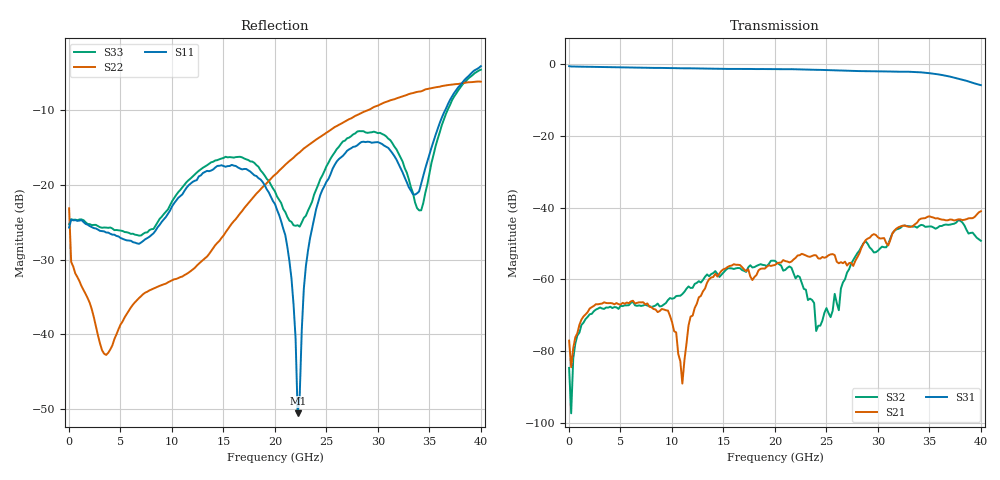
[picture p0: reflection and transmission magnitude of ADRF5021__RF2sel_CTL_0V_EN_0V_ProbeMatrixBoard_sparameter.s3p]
! Device:  ADRF5021
! Description: SOI MMIC SPDT Non-Reflective Switch
! Frequency:  9 kHz -  30 GHz
! Ports:
! 	RFC	= Port 1
!	RF1	= Port 2
!	RF2	= Port 3
! Vdd:  +3.3 Volt
! Vss:  -2.5 Volt
! Control:  0/+3.3 Volt
! State:  RF2 Selected (Vctl= 0 V, Ven= 0 V)
! Data:  The device was measured using G-S-G Probes on a matrix board.
!  Data was collected using an calibrated 4 port network analyzer.
!  The reference plane is the package pins of ADRF5021 switch.
! Note:  Analog Devices supplies this data as a sample of measured data at the package pin
!  for this product.  Your particular data for this product may vary.
!  Data was taken at 25 degrees C.
!  Analog Devices reserves the right to change this data at anytime.
# GHZ S DB R 50.0
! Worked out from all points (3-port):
!   201 points, 10 MHz to 40.01 GHz, reference 50 ohm
!   strongest paths, dB at 10 MHz, 10.01 GHz, 20.01 GHz, 30.01 GHz, 40.01 GHz:
!     S31: -0.6, -1.1, -1.4, -2.0, -5.9
!     S21: -77.1, -71.9, -56.0, -48.3, -41.0
!     S32: -84.7, -65.5, -54.9, -52.0, -49.3
!   lowest |S11| = -50.6 dB at 22.21 GHz (marker M1), VSWR 1.01, Z = 49.7 + j0.138 ohm
!   |S11| at or under -10 dB: start of sweep to 36.55 GHz
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0.01  -25.73 -14.1  -79.45 56.9  -0.58 0.3
      -77.11 -16.3  -23.15 79.6  -78.50 51.2
      -0.58 0.3  -84.72 -57.5  -25.27 -9.6
3.41  -26.24 -51.2  -66.72 32.8  -0.83 -40.4
      -66.43 34.1  -42.60 -166.9  -68.12 13.7
      -0.83 -40.4  -68.26 14.0  -25.72 -55.7
8.61  -25.68 -51.3  -69.35 19.9  -1.06 -100.7
      -69.15 18.3  -33.62 -94.7  -67.46 -56.8
      -1.05 -100.6  -66.78 -54.3  -24.99 -57.9
11.21  -20.83 -57.1  -81.36 -124.6  -1.18 -130.7
       -82.62 -137.9  -32.08 -73.6  -63.39 -109.7
       -1.18 -130.6  -63.49 -110.7  -19.99 -61.7
20.01  -22.58 -149.7  -55.96 102.3  -1.40 126.5
       -56.02 102.5  -18.66 -37.4  -54.87 65.2
       -1.40 126.6  -54.85 65.4  -20.90 -127.0
22.21  -50.57 152.2  -53.37 96.8  -1.46 99.7
       -53.37 96.4  -15.87 -41.9  -59.17 32.6
       -1.46 99.8  -59.02 32.0  -25.41 -87.7
25.61  -17.85 -38.1  -53.12 78.5  -1.75 57.9
       -52.99 78.5  -12.45 -53.2  -68.02 -114.2
       -1.73 58.0  -68.80 -110.3  -16.06 -53.0
28.81  -14.29 -72.4  -49.02 114.6  -1.97 18.9
       -49.10 115.7  -10.14 -66.0  -49.43 128.1
       -1.97 19.1  -49.39 129.3  -13.00 -81.1
34.21  -19.84 -41.3  -43.13 77.8  -2.31 -54.3
       -43.07 78.3  -7.50 -90.4  -44.72 71.5
       -2.31 -54.2  -44.84 72.2  -23.42 -49.8
40.01  -4.14 -68.0  -40.96 43.8  -5.87 -135.9
       -41.04 43.4  -6.21 -119.9  -49.69 27.8
       -5.87 -135.7  -49.27 28.4  -4.61 -52.0
